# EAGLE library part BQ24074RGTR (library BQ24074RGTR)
USB-Friendly Li-Ion Battery Charger and Power-Path Management IC, 10.5V OVP Source: Datasheet
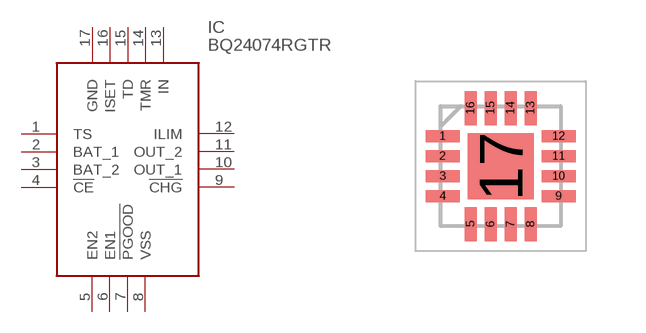
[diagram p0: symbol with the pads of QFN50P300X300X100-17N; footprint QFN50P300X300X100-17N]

Designator prefix IC

## BQ24074RGTR (Arrow_Part_Number: BQ24074RGTR; Arrow_Price-Stock: https://www.arrow.com/en/products/bq24074rgtr/texas-instruments?utm_currency=USD&region=nac; Description: USB-Friendly Li-Ion Battery Charger and Power-Path Management IC, 10.5V OVP; Height: 1mm; Manufacturer_Name: Texas Instruments; Manufacturer_Part_Number: BQ24074RGTR; Mouser_Part_Number: 595-BQ24074RGTR; Mouser_Price-Stock: https://www.mouser.co.uk/ProductDetail/Texas-Instruments/BQ24074RGTR?qs=ZV%2Fxhq4oszp2Nll7fIx5wg%3D%3D)  [QFN50P300X300X100-17N]
1  TS
2  BAT_1
3  BAT_2
4  !CE
5  EN2
6  EN1
7  !PGOOD
8  VSS
9  !CHG
10  OUT_1
11  OUT_2
12  ILIM
13  IN
14  TMR
15  TD
16  ISET
17  GND

## Footprint QFN50P300X300X100-17N (pad centres in mm)
BQ24074RGTR-1
smd 0.85 x 0.3: 1 -1.45,0.75; 2 -1.45,0.25; 3 -1.45,-0.25; 4 -1.45,-0.75; 9 1.45,-0.75; 10 1.45,-0.25; 11 1.45,0.25; 12 1.45,0.75
smd 0.3 x 0.85: 5 -0.75,-1.45; 6 -0.25,-1.45; 7 0.25,-1.45; 8 0.75,-1.45; 13 0.75,1.45; 14 0.25,1.45; 15 -0.25,1.45; 16 -0.75,1.45
smd 1.65 x 1.65: 17 0,0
